(* Logix 5000 Program export IO_Mapping; software revision 30.00; part 3 of 3 *)
(* tags used below, declared in another part *)
   L_INC : L_INC;
   TEMP : INT;
   DATA_MSG_NODE1 : VMAC_DATA_MSG;
   DATA_MSG_NODE3 : VMAC_DATA_MSG;
   DATA_MSG_NODE4 : VMAC_DATA_MSG;
   EdDSA_KS : DINT[8];
   EdDSA_KS_Prime : DINT[8];
   InternalFlag_AllNodesHaveMyKsPrime : BOOL;
   InternalFlag_KsID : LINT;
   InternalFlag_KsPrimeID : LINT;
   KAF_COMMS_UP : BOOL;   // TEMP TAG
   NODE : VMAC_DATA_INTERNAL[5];
   VMAC_KEY : DINT[8];
   VMAC_KEY_ID : LINT;
   Wrk_InpA : DINT[2];
   Wrk_InpB : DINT[2];
(* IO_Mapping, continued *)

ROUTINE VI_NODE3   (* ladder *)
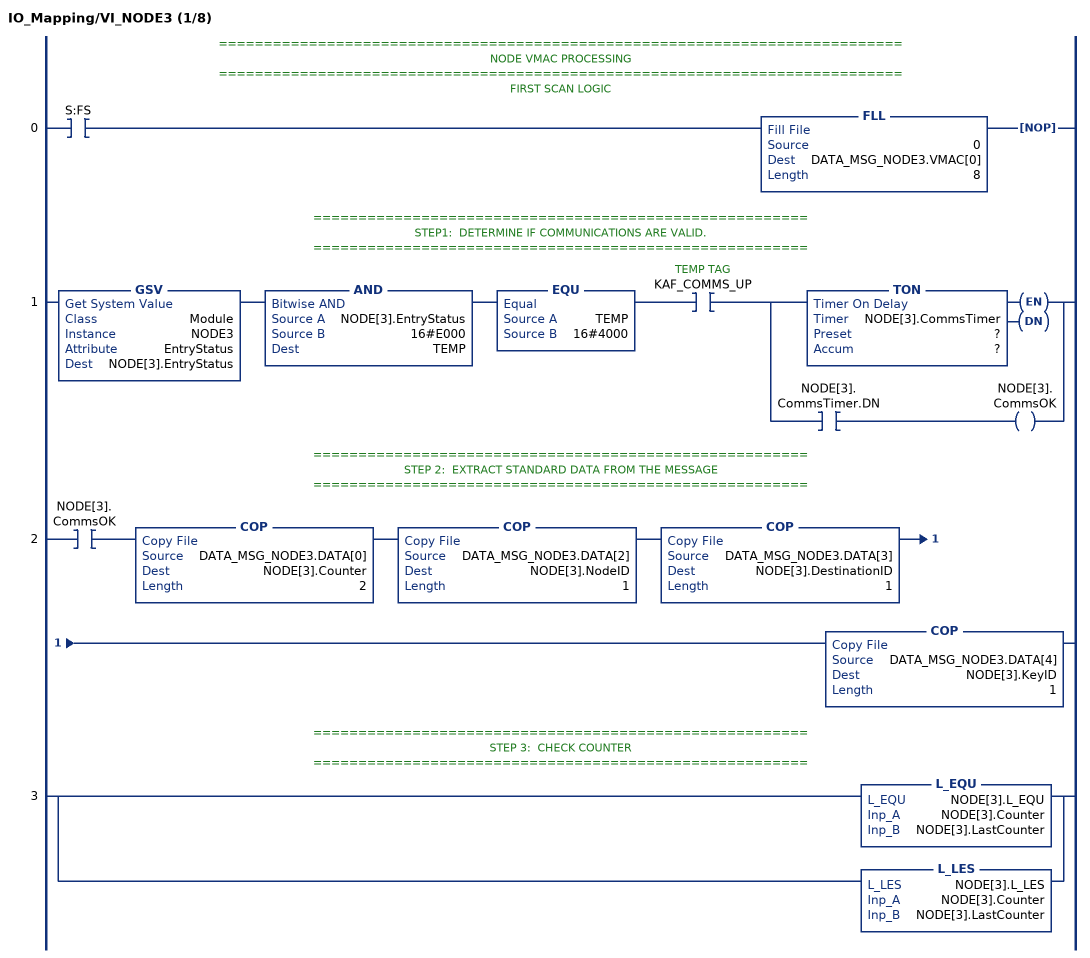
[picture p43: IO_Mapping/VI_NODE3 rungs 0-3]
   // ============================================================================
   // NODE VMAC PROCESSING
   // ============================================================================
   // FIRST SCAN LOGIC
   0: XIC(S:FS)FLL(0,DATA_MSG_NODE3.VMAC[0],8)NOP();
   // =======================================================
   // STEP1:  DETERMINE IF COMMUNICATIONS ARE VALID.
   // =======================================================
   1: GSV(Module,NODE3,EntryStatus,NODE[3].EntryStatus)AND(NODE[3].EntryStatus,16#E000,TEMP)EQU(TEMP,16#4000)XIC(KAF_COMMS_UP)[TON(NODE[3].CommsTimer,?,?) ,XIC(NODE[3].CommsTimer.DN) OTE(NODE[3].CommsOK) ];
   // =======================================================
   // STEP 2:  EXTRACT STANDARD DATA FROM THE MESSAGE
   // =======================================================
   2: XIC(NODE[3].CommsOK)COP(DATA_MSG_NODE3.DATA[0],NODE[3].Counter,2)COP(DATA_MSG_NODE3.DATA[2],NODE[3].NodeID,1)COP(DATA_MSG_NODE3.DATA[3],NODE[3].DestinationID,1)COP(DATA_MSG_NODE3.DATA[4],NODE[3].KeyID,1);
   // =======================================================
   // STEP 3:  CHECK COUNTER
   // =======================================================
   3: [L_EQU(NODE[3].L_EQU,NODE[3].Counter,NODE[3].LastCounter) ,L_LES(NODE[3].L_LES,NODE[3].Counter,NODE[3].LastCounter) ];
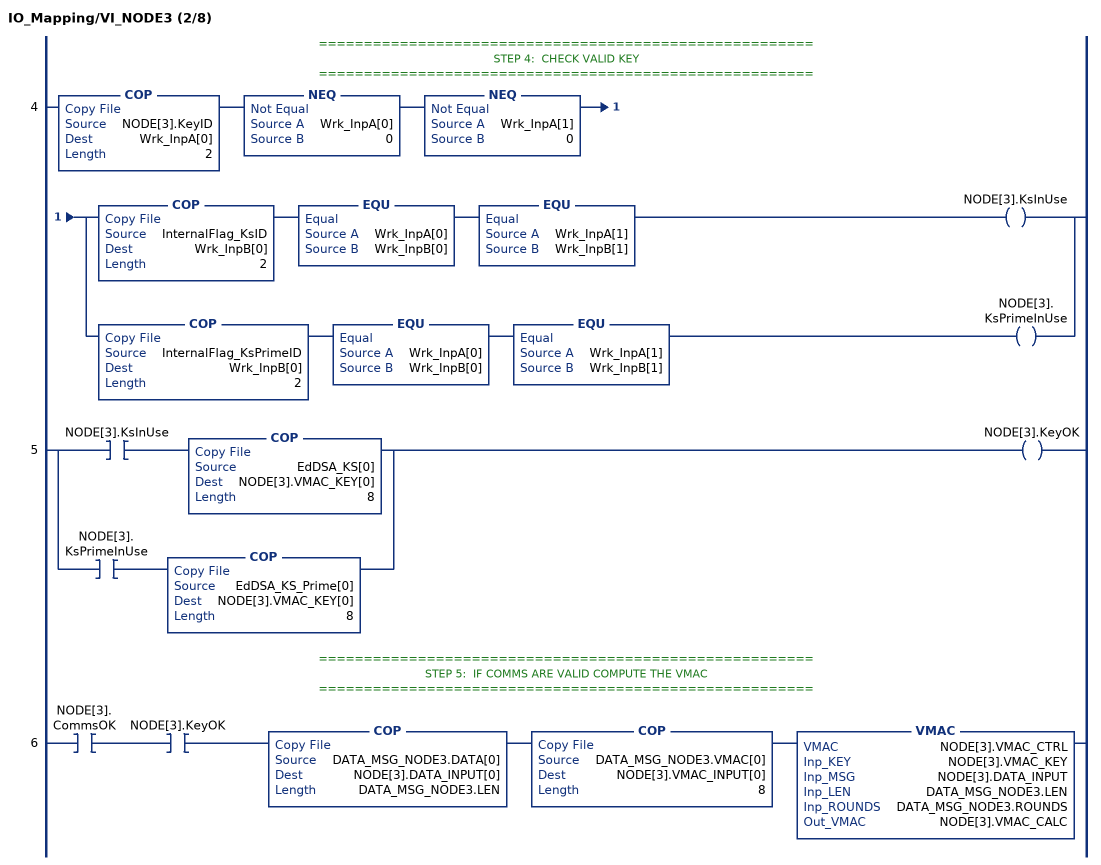
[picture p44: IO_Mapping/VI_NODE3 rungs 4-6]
   // =======================================================
   // STEP 4:  CHECK VALID KEY
   // =======================================================
   4: COP(NODE[3].KeyID,Wrk_InpA[0],2)NEQ(Wrk_InpA[0],0)NEQ(Wrk_InpA[1],0)[COP(InternalFlag_KsID,Wrk_InpB[0],2) EQU(Wrk_InpA[0],Wrk_InpB[0]) EQU(Wrk_InpA[1],Wrk_InpB[1]) OTE(NODE[3].KsInUse) ,COP(InternalFlag_KsPrimeID,Wrk_InpB[0],2) EQU(Wrk_InpA[0],Wrk_InpB[0]) EQU(Wrk_InpA[1],Wrk_InpB[1]) OTE(NODE[3].KsPrimeInUse) ];
   5: [XIC(NODE[3].KsInUse) COP(EdDSA_KS[0],NODE[3].VMAC_KEY[0],8) ,XIC(NODE[3].KsPrimeInUse) COP(EdDSA_KS_Prime[0],NODE[3].VMAC_KEY[0],8) ]OTE(NODE[3].KeyOK);
   // =======================================================
   // STEP 5:  IF COMMS ARE VALID COMPUTE THE VMAC
   // =======================================================
   6: XIC(NODE[3].CommsOK)XIC(NODE[3].KeyOK)COP(DATA_MSG_NODE3.DATA[0],NODE[3].DATA_INPUT[0],DATA_MSG_NODE3.LEN)COP(DATA_MSG_NODE3.VMAC[0],NODE[3].VMAC_INPUT[0],8)VMAC(NODE[3].VMAC_CTRL,NODE[3].VMAC_KEY,NODE[3].DATA_INPUT,DATA_MSG_NODE3.LEN,DATA_MSG_NODE3.ROUNDS,NODE[3].VMAC_CALC);
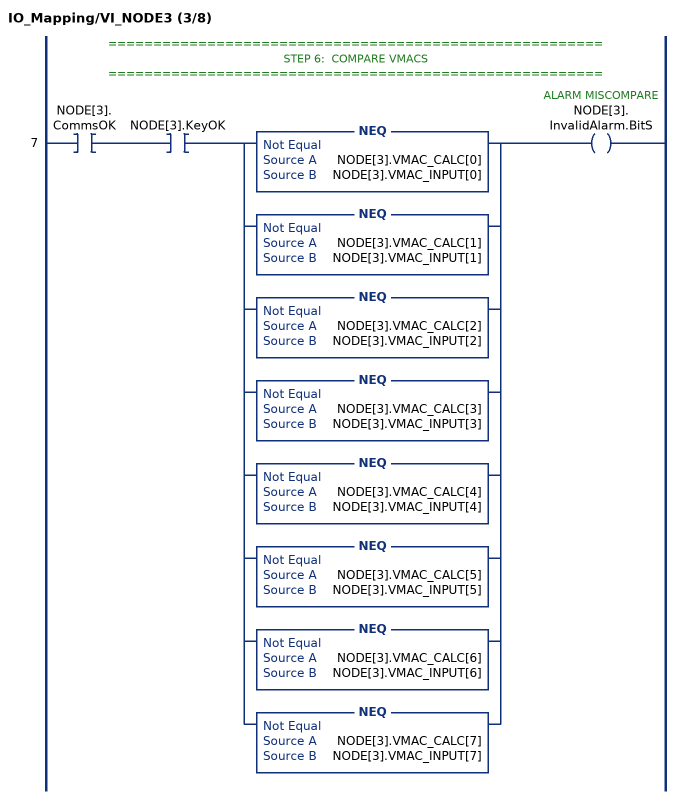
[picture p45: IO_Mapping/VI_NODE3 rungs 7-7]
   // =======================================================
   // STEP 6:  COMPARE VMACS
   // =======================================================
   7: XIC(NODE[3].CommsOK)XIC(NODE[3].KeyOK)[NEQ(NODE[3].VMAC_CALC[0],NODE[3].VMAC_INPUT[0]) ,NEQ(NODE[3].VMAC_CALC[1],NODE[3].VMAC_INPUT[1]) ,NEQ(NODE[3].VMAC_CALC[2],NODE[3].VMAC_INPUT[2]) ,NEQ(NODE[3].VMAC_CALC[3],NODE[3].VMAC_INPUT[3]) ,NEQ(NODE[3].VMAC_CALC[4],NODE[3].VMAC_INPUT[4]) ,NEQ(NODE[3].VMAC_CALC[5],NODE[3].VMAC_INPUT[5]) ,NEQ(NODE[3].VMAC_CALC[6],NODE[3].VMAC_INPUT[6]) ,NEQ(NODE[3].VMAC_CALC[7],NODE[3].VMAC_INPUT[7]) ]OTE(NODE[3].InvalidAlarm.BitS);
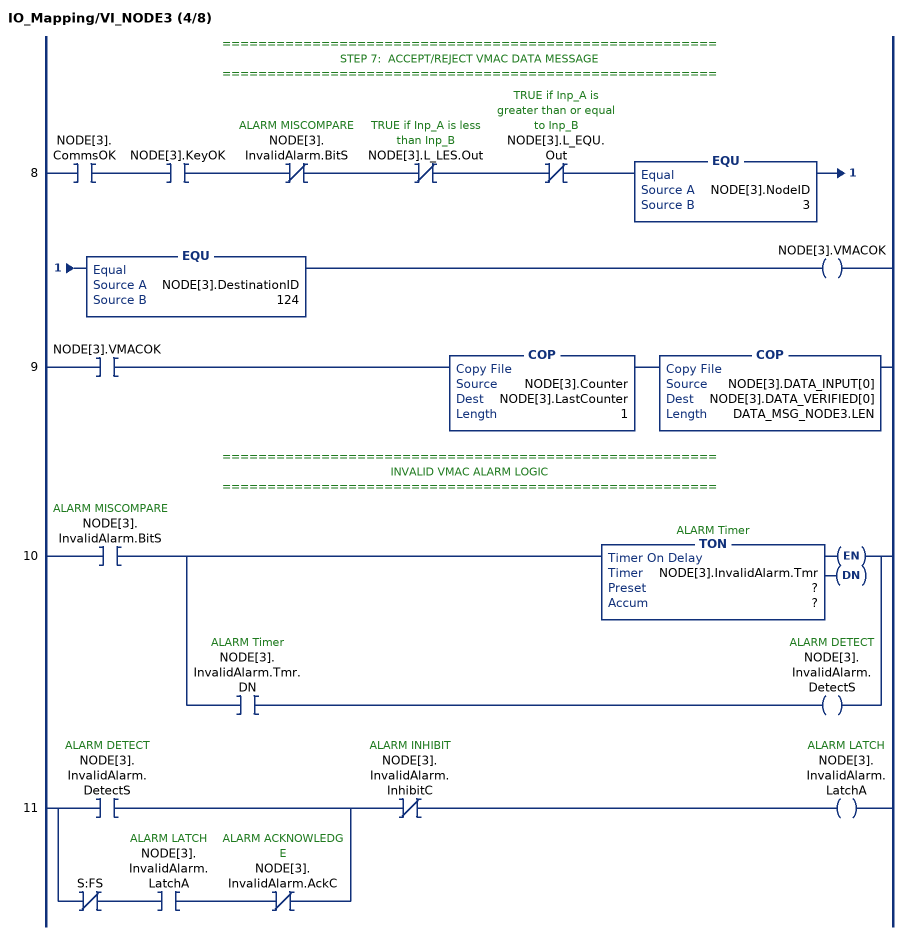
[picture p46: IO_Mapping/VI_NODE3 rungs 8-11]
   // =======================================================
   // STEP 7:  ACCEPT/REJECT VMAC DATA MESSAGE
   // =======================================================
   8: XIC(NODE[3].CommsOK)XIC(NODE[3].KeyOK)XIO(NODE[3].InvalidAlarm.BitS)XIO(NODE[3].L_LES.Out)XIO(NODE[3].L_EQU.Out)EQU(NODE[3].NodeID,3)EQU(NODE[3].DestinationID,124)OTE(NODE[3].VMACOK);
   9: XIC(NODE[3].VMACOK)COP(NODE[3].Counter,NODE[3].LastCounter,1)COP(NODE[3].DATA_INPUT[0],NODE[3].DATA_VERIFIED[0],DATA_MSG_NODE3.LEN);
   // =======================================================
   // INVALID VMAC ALARM LOGIC
   // =======================================================
   10: XIC(NODE[3].InvalidAlarm.BitS)[TON(NODE[3].InvalidAlarm.Tmr,?,?) ,XIC(NODE[3].InvalidAlarm.Tmr.DN) OTE(NODE[3].InvalidAlarm.DetectS) ];
   11: [XIC(NODE[3].InvalidAlarm.DetectS) ,XIO(S:FS) XIC(NODE[3].InvalidAlarm.LatchA) XIO(NODE[3].InvalidAlarm.AckC) ]XIO(NODE[3].InvalidAlarm.InhibitC)OTE(NODE[3].InvalidAlarm.LatchA);
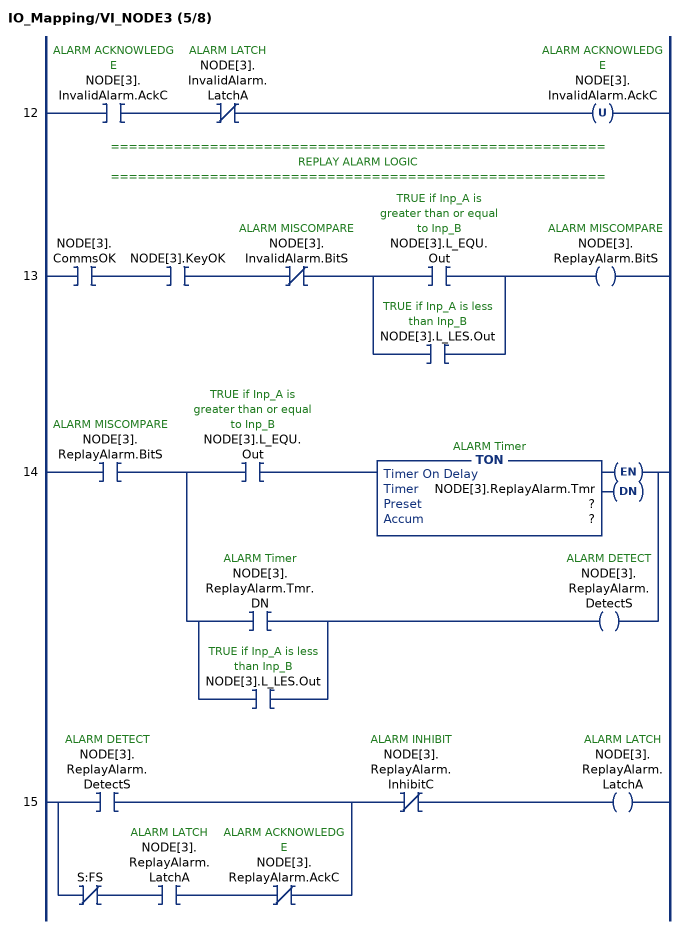
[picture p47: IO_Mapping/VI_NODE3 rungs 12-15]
   12: XIC(NODE[3].InvalidAlarm.AckC)XIO(NODE[3].InvalidAlarm.LatchA)OTU(NODE[3].InvalidAlarm.AckC);
   // =======================================================
   // REPLAY ALARM LOGIC
   // =======================================================
   13: XIC(NODE[3].CommsOK)XIC(NODE[3].KeyOK)XIO(NODE[3].InvalidAlarm.BitS)[XIC(NODE[3].L_EQU.Out) ,XIC(NODE[3].L_LES.Out) ]OTE(NODE[3].ReplayAlarm.BitS);
   14: XIC(NODE[3].ReplayAlarm.BitS)[XIC(NODE[3].L_EQU.Out) TON(NODE[3].ReplayAlarm.Tmr,?,?) ,[XIC(NODE[3].ReplayAlarm.Tmr.DN) ,XIC(NODE[3].L_LES.Out) ] OTE(NODE[3].ReplayAlarm.DetectS) ];
   15: [XIC(NODE[3].ReplayAlarm.DetectS) ,XIO(S:FS) XIC(NODE[3].ReplayAlarm.LatchA) XIO(NODE[3].ReplayAlarm.AckC) ]XIO(NODE[3].ReplayAlarm.InhibitC)OTE(NODE[3].ReplayAlarm.LatchA);
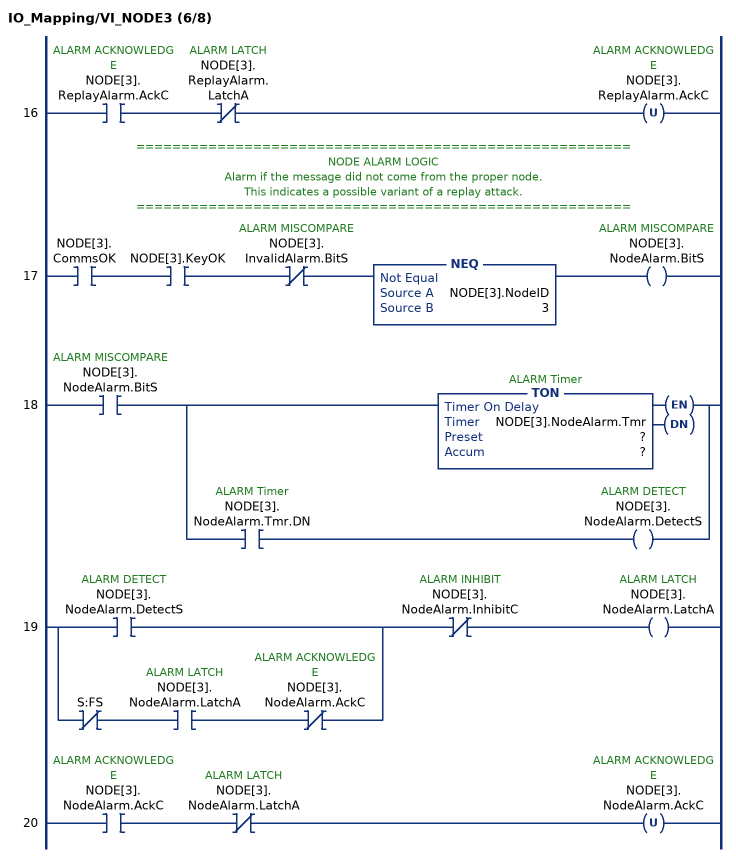
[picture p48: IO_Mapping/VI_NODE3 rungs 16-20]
   16: XIC(NODE[3].ReplayAlarm.AckC)XIO(NODE[3].ReplayAlarm.LatchA)OTU(NODE[3].ReplayAlarm.AckC);
   // =======================================================
   // NODE ALARM LOGIC
   // Alarm if the message did not come from the proper node.
   // This indicates a possible variant of a replay attack.
   // =======================================================
   17: XIC(NODE[3].CommsOK)XIC(NODE[3].KeyOK)XIO(NODE[3].InvalidAlarm.BitS)NEQ(NODE[3].NodeID,3)OTE(NODE[3].NodeAlarm.BitS);
   18: XIC(NODE[3].NodeAlarm.BitS)[TON(NODE[3].NodeAlarm.Tmr,?,?) ,XIC(NODE[3].NodeAlarm.Tmr.DN) OTE(NODE[3].NodeAlarm.DetectS) ];
   19: [XIC(NODE[3].NodeAlarm.DetectS) ,XIO(S:FS) XIC(NODE[3].NodeAlarm.LatchA) XIO(NODE[3].NodeAlarm.AckC) ]XIO(NODE[3].NodeAlarm.InhibitC)OTE(NODE[3].NodeAlarm.LatchA);
   20: XIC(NODE[3].NodeAlarm.AckC)XIO(NODE[3].NodeAlarm.LatchA)OTU(NODE[3].NodeAlarm.AckC);
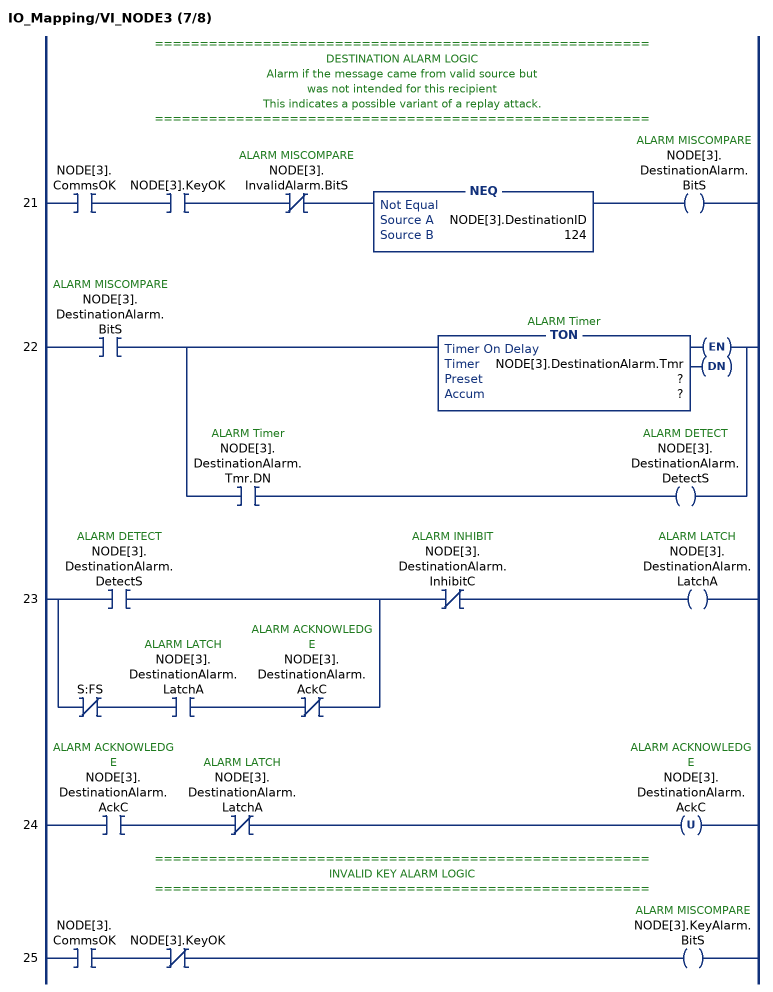
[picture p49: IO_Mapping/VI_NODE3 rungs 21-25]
   // =======================================================
   // DESTINATION ALARM LOGIC
   // Alarm if the message came from valid source but
   // was not intended for this recipient
   // This indicates a possible variant of a replay attack.
   // =======================================================
   21: XIC(NODE[3].CommsOK)XIC(NODE[3].KeyOK)XIO(NODE[3].InvalidAlarm.BitS)NEQ(NODE[3].DestinationID,124)OTE(NODE[3].DestinationAlarm.BitS);
   22: XIC(NODE[3].DestinationAlarm.BitS)[TON(NODE[3].DestinationAlarm.Tmr,?,?) ,XIC(NODE[3].DestinationAlarm.Tmr.DN) OTE(NODE[3].DestinationAlarm.DetectS) ];
   23: [XIC(NODE[3].DestinationAlarm.DetectS) ,XIO(S:FS) XIC(NODE[3].DestinationAlarm.LatchA) XIO(NODE[3].DestinationAlarm.AckC) ]XIO(NODE[3].DestinationAlarm.InhibitC)OTE(NODE[3].DestinationAlarm.LatchA);
   24: XIC(NODE[3].DestinationAlarm.AckC)XIO(NODE[3].DestinationAlarm.LatchA)OTU(NODE[3].DestinationAlarm.AckC);
   // =======================================================
   // INVALID KEY ALARM LOGIC
   // =======================================================
   25: XIC(NODE[3].CommsOK)XIO(NODE[3].KeyOK)OTE(NODE[3].KeyAlarm.BitS);
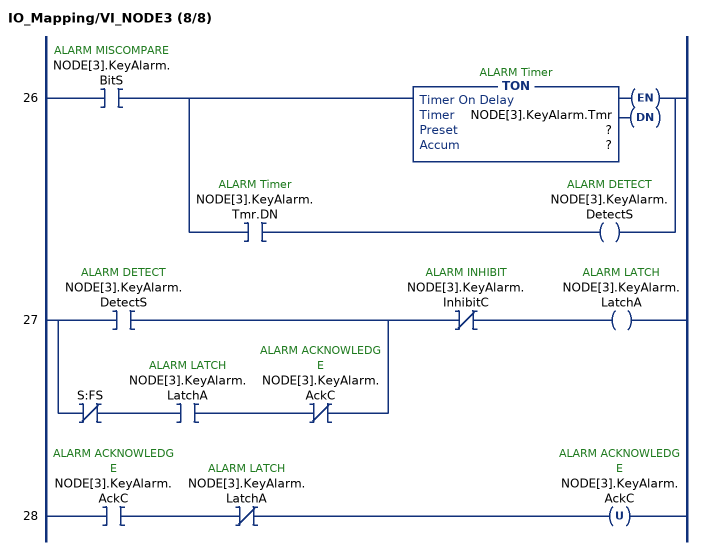
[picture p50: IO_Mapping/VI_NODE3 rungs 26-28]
   26: XIC(NODE[3].KeyAlarm.BitS)[TON(NODE[3].KeyAlarm.Tmr,?,?) ,XIC(NODE[3].KeyAlarm.Tmr.DN) OTE(NODE[3].KeyAlarm.DetectS) ];
   27: [XIC(NODE[3].KeyAlarm.DetectS) ,XIO(S:FS) XIC(NODE[3].KeyAlarm.LatchA) XIO(NODE[3].KeyAlarm.AckC) ]XIO(NODE[3].KeyAlarm.InhibitC)OTE(NODE[3].KeyAlarm.LatchA);
   28: XIC(NODE[3].KeyAlarm.AckC)XIO(NODE[3].KeyAlarm.LatchA)OTU(NODE[3].KeyAlarm.AckC);
END_ROUTINE

ROUTINE VI_NODE4   (* ladder *)
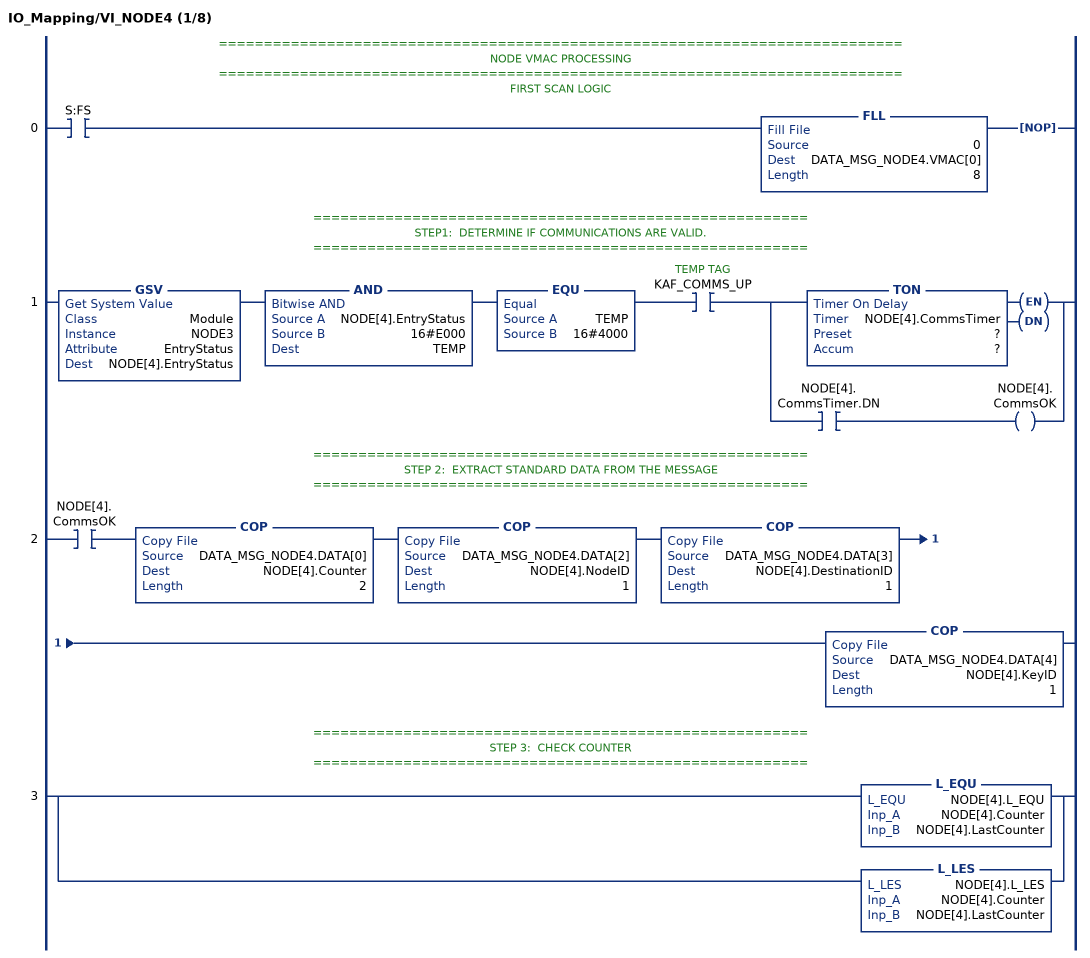
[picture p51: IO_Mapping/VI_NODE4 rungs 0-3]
   // ============================================================================
   // NODE VMAC PROCESSING
   // ============================================================================
   // FIRST SCAN LOGIC
   0: XIC(S:FS)FLL(0,DATA_MSG_NODE4.VMAC[0],8)NOP();
   // =======================================================
   // STEP1:  DETERMINE IF COMMUNICATIONS ARE VALID.
   // =======================================================
   1: GSV(Module,NODE3,EntryStatus,NODE[4].EntryStatus)AND(NODE[4].EntryStatus,16#E000,TEMP)EQU(TEMP,16#4000)XIC(KAF_COMMS_UP)[TON(NODE[4].CommsTimer,?,?) ,XIC(NODE[4].CommsTimer.DN) OTE(NODE[4].CommsOK) ];
   // =======================================================
   // STEP 2:  EXTRACT STANDARD DATA FROM THE MESSAGE
   // =======================================================
   2: XIC(NODE[4].CommsOK)COP(DATA_MSG_NODE4.DATA[0],NODE[4].Counter,2)COP(DATA_MSG_NODE4.DATA[2],NODE[4].NodeID,1)COP(DATA_MSG_NODE4.DATA[3],NODE[4].DestinationID,1)COP(DATA_MSG_NODE4.DATA[4],NODE[4].KeyID,1);
   // =======================================================
   // STEP 3:  CHECK COUNTER
   // =======================================================
   3: [L_EQU(NODE[4].L_EQU,NODE[4].Counter,NODE[4].LastCounter) ,L_LES(NODE[4].L_LES,NODE[4].Counter,NODE[4].LastCounter) ];
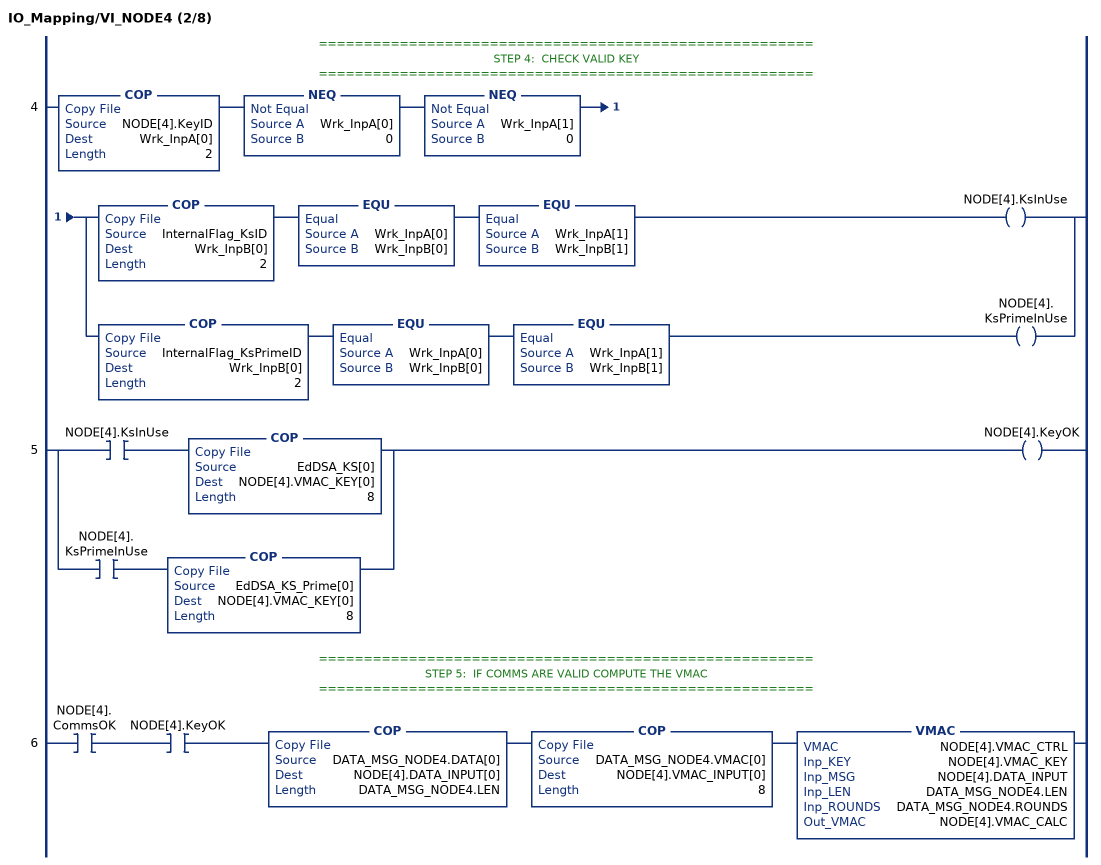
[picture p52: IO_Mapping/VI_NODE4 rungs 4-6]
   // =======================================================
   // STEP 4:  CHECK VALID KEY
   // =======================================================
   4: COP(NODE[4].KeyID,Wrk_InpA[0],2)NEQ(Wrk_InpA[0],0)NEQ(Wrk_InpA[1],0)[COP(InternalFlag_KsID,Wrk_InpB[0],2) EQU(Wrk_InpA[0],Wrk_InpB[0]) EQU(Wrk_InpA[1],Wrk_InpB[1]) OTE(NODE[4].KsInUse) ,COP(InternalFlag_KsPrimeID,Wrk_InpB[0],2) EQU(Wrk_InpA[0],Wrk_InpB[0]) EQU(Wrk_InpA[1],Wrk_InpB[1]) OTE(NODE[4].KsPrimeInUse) ];
   5: [XIC(NODE[4].KsInUse) COP(EdDSA_KS[0],NODE[4].VMAC_KEY[0],8) ,XIC(NODE[4].KsPrimeInUse) COP(EdDSA_KS_Prime[0],NODE[4].VMAC_KEY[0],8) ]OTE(NODE[4].KeyOK);
   // =======================================================
   // STEP 5:  IF COMMS ARE VALID COMPUTE THE VMAC
   // =======================================================
   6: XIC(NODE[4].CommsOK)XIC(NODE[4].KeyOK)COP(DATA_MSG_NODE4.DATA[0],NODE[4].DATA_INPUT[0],DATA_MSG_NODE4.LEN)COP(DATA_MSG_NODE4.VMAC[0],NODE[4].VMAC_INPUT[0],8)VMAC(NODE[4].VMAC_CTRL,NODE[4].VMAC_KEY,NODE[4].DATA_INPUT,DATA_MSG_NODE4.LEN,DATA_MSG_NODE4.ROUNDS,NODE[4].VMAC_CALC);
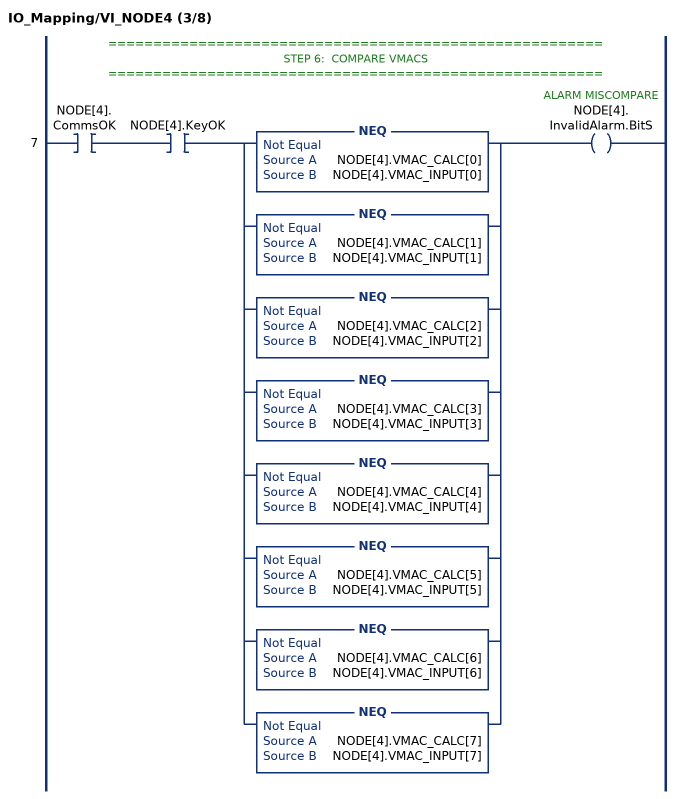
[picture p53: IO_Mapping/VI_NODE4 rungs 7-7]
   // =======================================================
   // STEP 6:  COMPARE VMACS
   // =======================================================
   7: XIC(NODE[4].CommsOK)XIC(NODE[4].KeyOK)[NEQ(NODE[4].VMAC_CALC[0],NODE[4].VMAC_INPUT[0]) ,NEQ(NODE[4].VMAC_CALC[1],NODE[4].VMAC_INPUT[1]) ,NEQ(NODE[4].VMAC_CALC[2],NODE[4].VMAC_INPUT[2]) ,NEQ(NODE[4].VMAC_CALC[3],NODE[4].VMAC_INPUT[3]) ,NEQ(NODE[4].VMAC_CALC[4],NODE[4].VMAC_INPUT[4]) ,NEQ(NODE[4].VMAC_CALC[5],NODE[4].VMAC_INPUT[5]) ,NEQ(NODE[4].VMAC_CALC[6],NODE[4].VMAC_INPUT[6]) ,NEQ(NODE[4].VMAC_CALC[7],NODE[4].VMAC_INPUT[7]) ]OTE(NODE[4].InvalidAlarm.BitS);
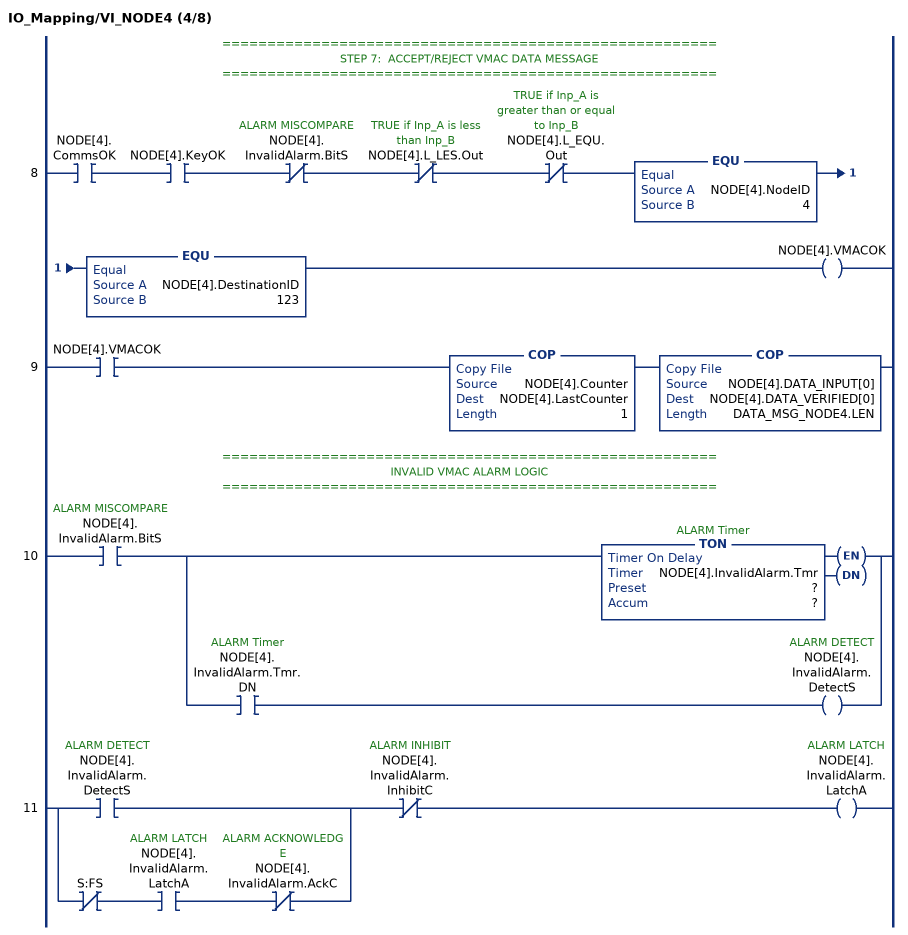
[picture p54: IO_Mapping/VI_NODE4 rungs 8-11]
   // =======================================================
   // STEP 7:  ACCEPT/REJECT VMAC DATA MESSAGE
   // =======================================================
   8: XIC(NODE[4].CommsOK)XIC(NODE[4].KeyOK)XIO(NODE[4].InvalidAlarm.BitS)XIO(NODE[4].L_LES.Out)XIO(NODE[4].L_EQU.Out)EQU(NODE[4].NodeID,4)EQU(NODE[4].DestinationID,123)OTE(NODE[4].VMACOK);
   9: XIC(NODE[4].VMACOK)COP(NODE[4].Counter,NODE[4].LastCounter,1)COP(NODE[4].DATA_INPUT[0],NODE[4].DATA_VERIFIED[0],DATA_MSG_NODE4.LEN);
   // =======================================================
   // INVALID VMAC ALARM LOGIC
   // =======================================================
   10: XIC(NODE[4].InvalidAlarm.BitS)[TON(NODE[4].InvalidAlarm.Tmr,?,?) ,XIC(NODE[4].InvalidAlarm.Tmr.DN) OTE(NODE[4].InvalidAlarm.DetectS) ];
   11: [XIC(NODE[4].InvalidAlarm.DetectS) ,XIO(S:FS) XIC(NODE[4].InvalidAlarm.LatchA) XIO(NODE[4].InvalidAlarm.AckC) ]XIO(NODE[4].InvalidAlarm.InhibitC)OTE(NODE[4].InvalidAlarm.LatchA);
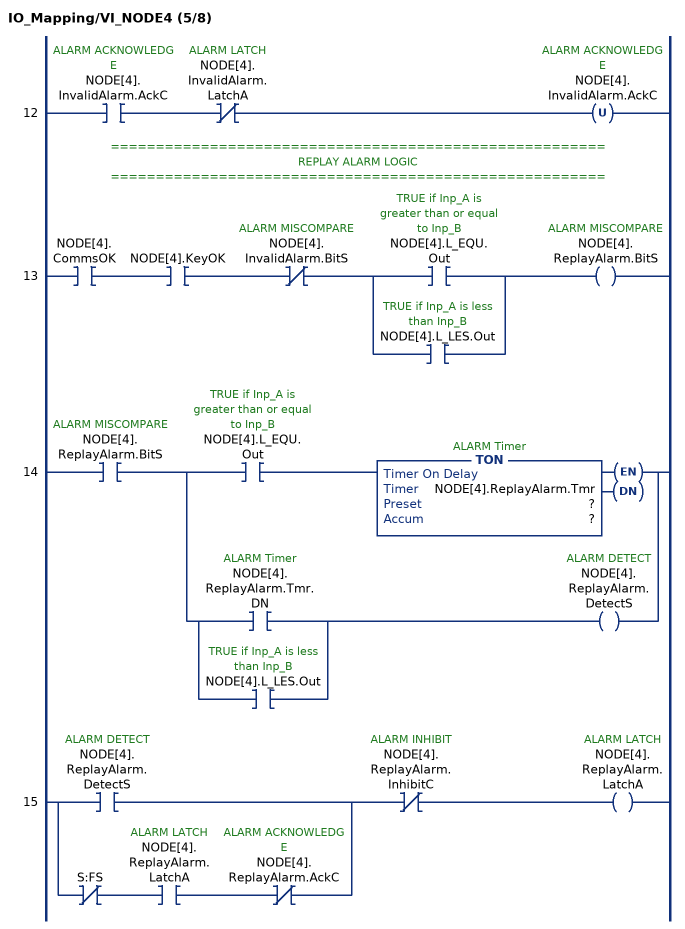
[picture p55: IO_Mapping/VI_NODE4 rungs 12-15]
   12: XIC(NODE[4].InvalidAlarm.AckC)XIO(NODE[4].InvalidAlarm.LatchA)OTU(NODE[4].InvalidAlarm.AckC);
   // =======================================================
   // REPLAY ALARM LOGIC
   // =======================================================
   13: XIC(NODE[4].CommsOK)XIC(NODE[4].KeyOK)XIO(NODE[4].InvalidAlarm.BitS)[XIC(NODE[4].L_EQU.Out) ,XIC(NODE[4].L_LES.Out) ]OTE(NODE[4].ReplayAlarm.BitS);
   14: XIC(NODE[4].ReplayAlarm.BitS)[XIC(NODE[4].L_EQU.Out) TON(NODE[4].ReplayAlarm.Tmr,?,?) ,[XIC(NODE[4].ReplayAlarm.Tmr.DN) ,XIC(NODE[4].L_LES.Out) ] OTE(NODE[4].ReplayAlarm.DetectS) ];
   15: [XIC(NODE[4].ReplayAlarm.DetectS) ,XIO(S:FS) XIC(NODE[4].ReplayAlarm.LatchA) XIO(NODE[4].ReplayAlarm.AckC) ]XIO(NODE[4].ReplayAlarm.InhibitC)OTE(NODE[4].ReplayAlarm.LatchA);
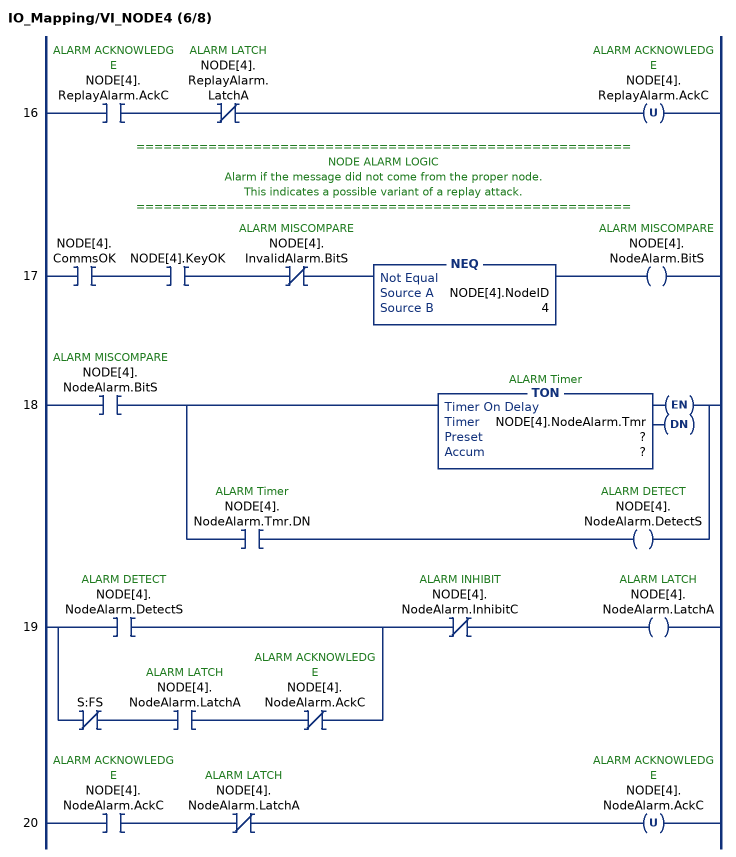
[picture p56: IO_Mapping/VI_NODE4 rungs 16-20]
   16: XIC(NODE[4].ReplayAlarm.AckC)XIO(NODE[4].ReplayAlarm.LatchA)OTU(NODE[4].ReplayAlarm.AckC);
   // =======================================================
   // NODE ALARM LOGIC
   // Alarm if the message did not come from the proper node.
   // This indicates a possible variant of a replay attack.
   // =======================================================
   17: XIC(NODE[4].CommsOK)XIC(NODE[4].KeyOK)XIO(NODE[4].InvalidAlarm.BitS)NEQ(NODE[4].NodeID,4)OTE(NODE[4].NodeAlarm.BitS);
   18: XIC(NODE[4].NodeAlarm.BitS)[TON(NODE[4].NodeAlarm.Tmr,?,?) ,XIC(NODE[4].NodeAlarm.Tmr.DN) OTE(NODE[4].NodeAlarm.DetectS) ];
   19: [XIC(NODE[4].NodeAlarm.DetectS) ,XIO(S:FS) XIC(NODE[4].NodeAlarm.LatchA) XIO(NODE[4].NodeAlarm.AckC) ]XIO(NODE[4].NodeAlarm.InhibitC)OTE(NODE[4].NodeAlarm.LatchA);
   20: XIC(NODE[4].NodeAlarm.AckC)XIO(NODE[4].NodeAlarm.LatchA)OTU(NODE[4].NodeAlarm.AckC);
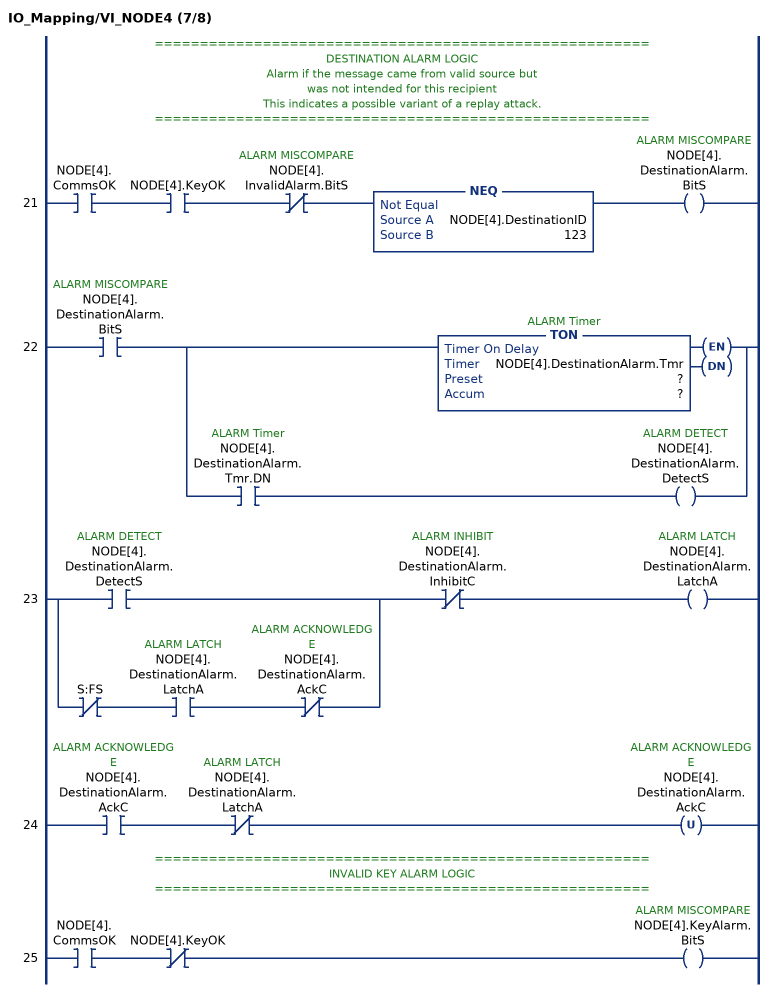
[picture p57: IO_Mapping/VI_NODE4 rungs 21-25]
   // =======================================================
   // DESTINATION ALARM LOGIC
   // Alarm if the message came from valid source but
   // was not intended for this recipient
   // This indicates a possible variant of a replay attack.
   // =======================================================
   21: XIC(NODE[4].CommsOK)XIC(NODE[4].KeyOK)XIO(NODE[4].InvalidAlarm.BitS)NEQ(NODE[4].DestinationID,123)OTE(NODE[4].DestinationAlarm.BitS);
   22: XIC(NODE[4].DestinationAlarm.BitS)[TON(NODE[4].DestinationAlarm.Tmr,?,?) ,XIC(NODE[4].DestinationAlarm.Tmr.DN) OTE(NODE[4].DestinationAlarm.DetectS) ];
   23: [XIC(NODE[4].DestinationAlarm.DetectS) ,XIO(S:FS) XIC(NODE[4].DestinationAlarm.LatchA) XIO(NODE[4].DestinationAlarm.AckC) ]XIO(NODE[4].DestinationAlarm.InhibitC)OTE(NODE[4].DestinationAlarm.LatchA);
   24: XIC(NODE[4].DestinationAlarm.AckC)XIO(NODE[4].DestinationAlarm.LatchA)OTU(NODE[4].DestinationAlarm.AckC);
   // =======================================================
   // INVALID KEY ALARM LOGIC
   // =======================================================
   25: XIC(NODE[4].CommsOK)XIO(NODE[4].KeyOK)OTE(NODE[4].KeyAlarm.BitS);
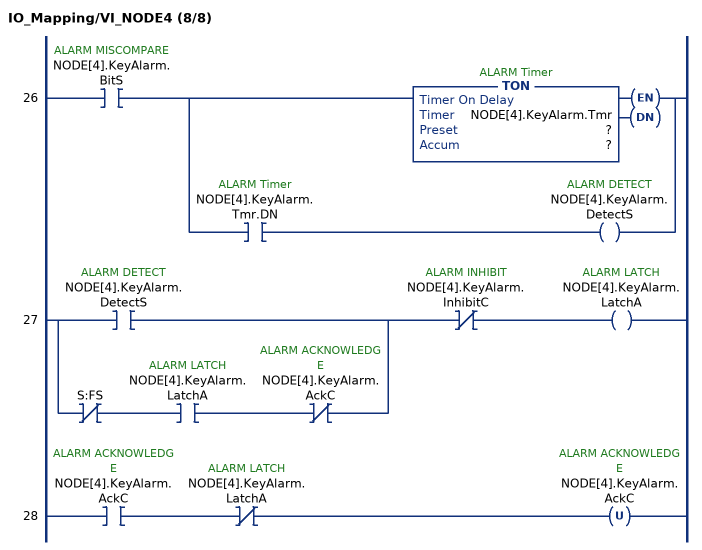
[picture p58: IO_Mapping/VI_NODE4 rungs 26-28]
   26: XIC(NODE[4].KeyAlarm.BitS)[TON(NODE[4].KeyAlarm.Tmr,?,?) ,XIC(NODE[4].KeyAlarm.Tmr.DN) OTE(NODE[4].KeyAlarm.DetectS) ];
   27: [XIC(NODE[4].KeyAlarm.DetectS) ,XIO(S:FS) XIC(NODE[4].KeyAlarm.LatchA) XIO(NODE[4].KeyAlarm.AckC) ]XIO(NODE[4].KeyAlarm.InhibitC)OTE(NODE[4].KeyAlarm.LatchA);
   28: XIC(NODE[4].KeyAlarm.AckC)XIO(NODE[4].KeyAlarm.LatchA)OTU(NODE[4].KeyAlarm.AckC);
END_ROUTINE

ROUTINE VO_NODE1   (* ladder *)
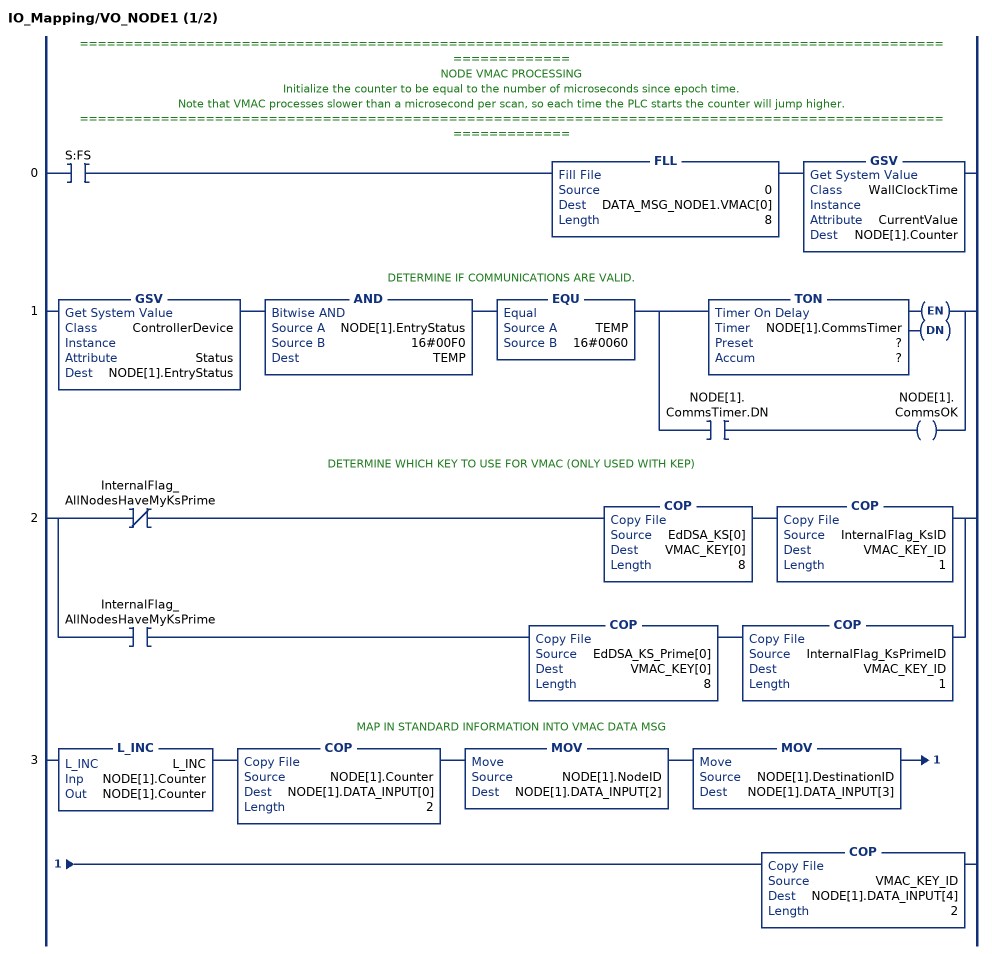
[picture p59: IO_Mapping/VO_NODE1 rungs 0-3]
   // =============================================================================================================
   // NODE VMAC PROCESSING
   // Initialize the counter to be equal to the number of microseconds since epoch time.
   // Note that VMAC processes slower than a microsecond per scan, so each time the PLC starts the counter will jump higher.
   // =============================================================================================================
   0: XIC(S:FS)FLL(0,DATA_MSG_NODE1.VMAC[0],8)GSV(WallClockTime,,CurrentValue,NODE[1].Counter);
   // DETERMINE IF COMMUNICATIONS ARE VALID.
   1: GSV(ControllerDevice,,Status,NODE[1].EntryStatus)AND(NODE[1].EntryStatus,16#00F0,TEMP)EQU(TEMP,16#0060)[TON(NODE[1].CommsTimer,?,?) ,XIC(NODE[1].CommsTimer.DN) OTE(NODE[1].CommsOK) ];
   // DETERMINE WHICH KEY TO USE FOR VMAC (ONLY USED WITH KEP)
   2: [XIO(InternalFlag_AllNodesHaveMyKsPrime) COP(EdDSA_KS[0],VMAC_KEY[0],8) COP(InternalFlag_KsID,VMAC_KEY_ID,1) ,XIC(InternalFlag_AllNodesHaveMyKsPrime) COP(EdDSA_KS_Prime[0],VMAC_KEY[0],8) COP(InternalFlag_KsPrimeID,VMAC_KEY_ID,1) ];
   // MAP IN STANDARD INFORMATION INTO VMAC DATA MSG
   3: L_INC(L_INC,NODE[1].Counter,NODE[1].Counter)COP(NODE[1].Counter,NODE[1].DATA_INPUT[0],2)MOV(NODE[1].NodeID,NODE[1].DATA_INPUT[2])MOV(NODE[1].DestinationID,NODE[1].DATA_INPUT[3])COP(VMAC_KEY_ID,NODE[1].DATA_INPUT[4],2);
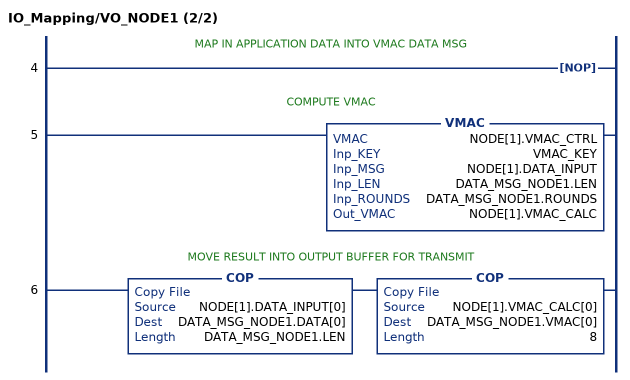
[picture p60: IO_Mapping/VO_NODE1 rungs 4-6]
   // MAP IN APPLICATION DATA INTO VMAC DATA MSG
   4: NOP();
   // COMPUTE VMAC
   5: VMAC(NODE[1].VMAC_CTRL,VMAC_KEY,NODE[1].DATA_INPUT,DATA_MSG_NODE1.LEN,DATA_MSG_NODE1.ROUNDS,NODE[1].VMAC_CALC);
   // MOVE RESULT INTO OUTPUT BUFFER FOR TRANSMIT
   6: COP(NODE[1].DATA_INPUT[0],DATA_MSG_NODE1.DATA[0],DATA_MSG_NODE1.LEN)COP(NODE[1].VMAC_CALC[0],DATA_MSG_NODE1.VMAC[0],8);
END_ROUTINE
END_PROGRAM
